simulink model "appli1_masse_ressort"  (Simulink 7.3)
settings: Solver=ode15s  StartTime=0.0  StopTime=1.0  RelTol=1e-3
StopFcn:
  | close all
  | load pos_vit.mat
  | plotyy(pv(1,:),pv(2,:),pv(1,:),pv(3,:))
  | gtext('Vitesse en ms/s')
  | gtext('Position en m')
  | grid
libraries: fl_lib x5, nesl_utility x3

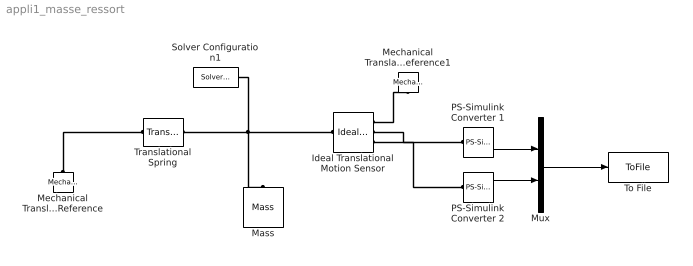
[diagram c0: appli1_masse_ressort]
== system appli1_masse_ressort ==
  Ideal Translational Motion Sensor : fl_lib/Mechanical/Mechanical Sensors/Ideal Translational Motion Sensor  DialogController=NetworkEngine.DynNeDlgSource  SystemSampleTime=-1  offset=0 m  v_Log=off  f_Log=off  x_Log=off  LocalVarNames=|v|f|x  LocalVarDescs=|v|f|x  LocalVarLogging=[0 0 0]
  Mass : fl_lib/Mechanical/Translational Elements/Mass  DialogController=NetworkEngine.DynNeDlgSource  SystemSampleTime=-1  mass=1 kg  initial_velocity=10 m/s  f_Log=off  LocalVarNames=|f  LocalVarDescs=|f  LocalVarLogging=0
  Mechanical Translational Reference : fl_lib/Mechanical/Translational Elements/Mechanical Translational Reference  DialogController=NetworkEngine.DynNeDlgSource  SystemSampleTime=-1  f_Log=off  LocalVarNames=|f  LocalVarDescs=|f  LocalVarLogging=0
  Mechanical Translational Reference1 : fl_lib/Mechanical/Translational Elements/Mechanical Translational Reference  DialogController=NetworkEngine.DynNeDlgSource  SystemSampleTime=-1  f_Log=off  LocalVarNames=|f  LocalVarDescs=|f  LocalVarLogging=0
  Mux : Mux  Inputs=2
  PS-Simulink Converter 1 : nesl_utility/PS-Simulink Converter  DialogController=NetworkEngine.DynNeUtilDlgSource  SystemSampleTime=-1  PhysicalDomain=network_engine_domain  LeftPortType=input  RightPortType=output  SubClassName=ps_output  Unit=m/s  AffineConversion=off
  PS-Simulink Converter 2 : nesl_utility/PS-Simulink Converter  DialogController=NetworkEngine.DynNeUtilDlgSource  SystemSampleTime=-1  PhysicalDomain=network_engine_domain  LeftPortType=input  RightPortType=output  SubClassName=ps_output  Unit=m  AffineConversion=off
  Solver Configuration1 : nesl_utility/Solver Configuration  DialogController=NetworkEngine.DynNeUtilDlgSource  SystemSampleTime=-1  PhysicalDomain=network_engine_domain  LeftPortType=input  RightPortType=generic  SubClassName=solver  Accelerate=off  Profile=off  ResidualTolerance=1e-9  MaxNonlinIter=12  MaxModeIter=2  DoFixedCost=off  DoDC=off  LinearAlgebra=Sparse
  To File : ToFile  Filename=pos_vit.mat  MatrixName=pv
  Translational Spring : fl_lib/Mechanical/Translational Elements/Translational Spring  DialogController=NetworkEngine.DynNeDlgSource  SystemSampleTime=-1  spr_rate=1000 N/m  init_def=0 m  f_Log=off  v_Log=off  x_Log=off  LocalVarNames=|f|v|x  LocalVarDescs=|f|v|x  LocalVarLogging=[0 0 0]
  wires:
  PS-Simulink Converter 1/1 -> Mux/1
  PS-Simulink Converter 2/1 -> Mux/2
  Mux/1 -> To File/1
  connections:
  Translational Spring/RConn1 -- Mass/LConn1 -- Ideal Translational Motion Sensor/LConn1 -- Solver Configuration1/RConn1
  Mechanical Translational Reference/LConn1 -- Translational Spring/LConn1
  Ideal Translational Motion Sensor/RConn1 -- Mechanical Translational Reference1/LConn1
  Ideal Translational Motion Sensor/RConn2 -- PS-Simulink Converter 1/LConn1
  Ideal Translational Motion Sensor/RConn3 -- PS-Simulink Converter 2/LConn1
